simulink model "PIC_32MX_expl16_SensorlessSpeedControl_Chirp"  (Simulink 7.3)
settings: Solver=FixedStepDiscrete  StartTime=0.0  StopTime=10.0  FixedStep=.002  RelTol=1e-3
undefined symbols (not defined in the file or in its folder): bits, Buffer, characters, contain, Cosine, DiscIntNeverNeededParam, full, is, OC_HW, OCmax, PWM, Receive, Sine, sl_helperblocks, slDataTypeAndScale, Timer3, uint, When
libraries: dsPICdrivers x8, simulink x7

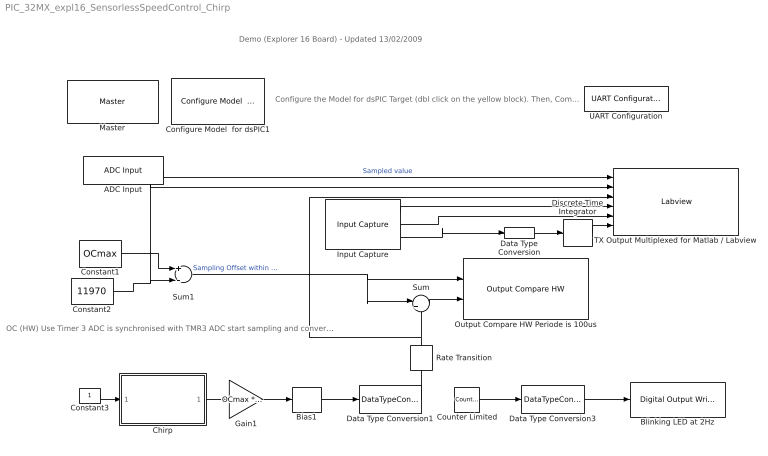
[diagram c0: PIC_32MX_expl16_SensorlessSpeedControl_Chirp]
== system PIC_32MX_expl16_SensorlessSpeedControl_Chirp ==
  note: Demo (Explorer 16 Board) - Updated 13/02/2009
  note: Configure the Model for dsPIC Target (dbl click on the yellow block). Then, Compile using the incremental build icon (second icon on right of the simulation mode (Normal))
  note: OC (HW) Use Timer 3 ADC is synchronised with TMR3 ADC start sampling and converting when TMR3 = OCmax (=PR3)
  ADC Input : dsPICdrivers/Peripheral I//O/ADC Input  Tag=dsPIC_ADC  Priority=5  ADC_TYPE=10 bits  ADC_MODE=Continuous sampling & get last channel value  NbrSampleStep=1  VoltRefpopup="AVdd  -  AVss"  OutFormatBitspopup=0000 00dd dddd dddd : Integer  InterruptPriority=6  ANCHANNELS=5  MaxName=ANmax = 1023  Rin=5e6  ADCS=29  SAMC=31  Temperature=25  DMAChannel=0  SampleTime=.002  Status="OK  |  Tsmp=4.844e-006 |  T/Channel=6.719e-006 |  Tall=6.719e-006"  SSRC=Timer3 (OC_HW PWM)
  Bias1 : Bias  Bias=floor(OCmax/2)
  Blinking LED at 2Hz : dsPICdrivers/Digital I//O/Digital Output Write  Tag=dsPIC_Digital_Output  Priority=5  PORT=A  Pin=[2]  Simultaneous=off  OrderingInOutPopup=None
  Chirp : Subsystem  mask{Fmax=15, Tend=60, Fs=500}
  Configure Model  for dsPIC1 : dsPICdrivers/Simulink Configuration/Configure Model  for dsPIC
  Constant1 : Constant  Value=OCmax  OutDataTypeMode=uint16  OutDataType=sfix(16)  OutScaling=2^0  OutDataTypeStr=uint16
  Constant2 : Constant  Value=11970  OutDataTypeMode=uint16  OutDataType=sfix(16)  OutScaling=2^0  OutDataTypeStr=uint16
  Constant3 : Constant  OutDataTypeMode=uint16  OutDataType=sfix(16)  OutScaling=2^0  OutDataTypeStr=uint16
  Counter Limited : simulink/Sources/Counter Limited  SystemSampleTime=-1  uplimit=1  tsamp=.25
  Data Type Conversion : DataTypeConversion  OutDataTypeMode=uint16  OutDataType=sfix(16)  OutScaling=2^0  OutDataTypeStr=uint16
  Data Type Conversion1 : DataTypeConversion  OutDataTypeMode=uint16  OutDataType=sfix(16)  OutScaling=2^0  OutDataTypeStr=uint16
  Data Type Conversion3 : DataTypeConversion  OutDataTypeMode=boolean  OutDataType=sfix(16)  OutScaling=2^0  OutDataTypeStr=boolean
  Discrete-Time Integrator : DiscreteIntegrator  gainval=500  SampleTime=-1  OutDataTypeMode=uint16  OutDataType=sfix(16)  OutScaling=2^0  OutDataTypeStr=uint16  ICPrevOutput=DiscIntNeverNeededParam  ICPrevScaledInput=DiscIntNeverNeededParam
  Gain1 : Gain  Gain=OCmax *.3  ParameterDataType=sfix(16)  ParameterScaling=2^0  OutDataTypeMode=int16  OutDataType=sfix(16)  OutScaling=2^0  OutDataTypeStr=int16
  Input Capture : dsPICdrivers/Peripheral I//O/Input Capture  Tag=dsPIC_PWM_IC  Priority=5  IntPriority=7  Channel=[1 ]  Channel_UP_Down_Periode=[3]  MaxChannel=[0.15]  SafeMarge=[10]  MaxName=' IC1max '  Precision=[15.917]  Timer=[2]  ChangeDetected=[1]  ChangeDetectedPortRef=3  SampleTime=-1  Status=OK
  Master : dsPICdrivers/Master  Tag=dsPIC_MASTER  Priority=1  TimeStepType=Timer1  picType=32MX460F512L  fcy=96000000  Quartz_33f=8e6  PLLActive_33f=on  fcyDesired_33f=96e6  tmr1="[8  23999  0]"  tmr1Info="Time Step : 0.002  ;   Error : 0%  PR1=23999"  tmr2345="[256    8    0    0]"  tmr2345cfg=[-1 -1 -1 -1]  IOautoConf=on  typePort="[ 0   0  10   0   0   0   0   0   0   0   0   0   0   0   0   0   0   0   0   0   0   8   0   0   0   0   0   0   0   0   0   0   0   0   0   0   0   0   0   0   0   0   0   0   0   0   0   0  24   0   0   0   0   0   0   0   6   0   0   0   0   0   0   0   0   0   0   0   0   0   0   0   0   0   0   0   0   0   0   0   0   0   0   0   4   5   0   0   0   0   0   0   0   0   0   0   0   0   0   0 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"  TRIS="[ 65531  65535  65535  65534  65535  65535  65535 ]"  ADPCFG=0  MasterBusyPort=None  MasterOverloadPort=None  FOSC=Quartz (XT - HS)  ClockSwitchMonitor=Both disabled  TempProtection_33f=TEMP_ON  FPBOR=<empty>  PWRT=disable  MCLR=<empty>  PowerSave=off  OverrideFcy=off  NewFcy=1e6  PR2345="[65535  11999  65535  65535]"
  Output Compare HW Periode is 100us : dsPICdrivers/Peripheral I//O/Output Compare HW  Tag=dsPIC_OC_HW_out  Priority=5  OC_Mode=PWM Time Set-Reset (glitch possible)  Timer=3  CHANNEL=[1 ]  Channel_UP_Down_Periode=[16]  PeriodeInput=off  MaxChannel=0.001  MaxName=' OCmax '  Precision=[13.5507]  Status=OK  SafeMarge=[0]  PortLetter=[68]  PortNumber=[0]  MaxValues=[11999]  NPORTS=2
  Rate Transition : RateTransition  Integrity=off
  Sum : Sum  Inputs=|++  OutDataType=sfix(16)  OutScaling=2^0
  Sum1 : Sum  Inputs=+-  OutDataType=sfix(16)  OutScaling=2^0
  TX Output Multiplexed for Matlab / Labview : dsPICdrivers/Serial PORT/TX Output Multiplexed for Matlab // Labview  Tag=dsPIC_TX_Multiplexed  Priority=5  UART=2  CleverSpreadingChk=on  CleverSpreading=1  CHANNEL=[0 1 2 3 4 5]  CHANNELBLOCKED=[]  CHANNELBLOCKED_BITEWISE=0  Status=OK
  UART Configuration : dsPICdrivers/Serial PORT/UART Configuration  Tag=dsPIC_config_UART  Priority=2  UART=2  proposed_BAUD=115200  ALT_TX_RX=on  InterruptTxWhen=When Transmit Buffer is empty  TXInterruptPri=1  TxBufferSize=32  TXEN=on  InterruptRxWhen=When Receive Buffer is full (contain 4 characters)  RXInterruptPri=2  RxBufferSize=32  BAUD=115200  UxBRG=51  Info="UxBRG = 51   ||  Real Baud : 115385   ||  % error : 0.16026  ||  max 23.0769 Bytes / Step"  RealBaud=0
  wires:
  Counter Limited/1 -> Data Type Conversion3/1
  ADC Input/1 -> TX Output Multiplexed for Matlab / Labview/1  "Sampled value"
  Sum/1 -> Output Compare HW Periode is 100us/2
  Sum1/1 -> Output Compare HW Periode is 100us/1, Sum/1  "Sampling Offset within PWM"
  Constant1/1 -> Sum1/1
  Data Type Conversion3/1 -> Blinking LED at 2Hz/1
  Rate Transition/1 -> Sum/2, TX Output Multiplexed for Matlab / Labview/3
  Input Capture/1 -> TX Output Multiplexed for Matlab / Labview/4
  Input Capture/2 -> TX Output Multiplexed for Matlab / Labview/5
  Input Capture/3 -> Data Type Conversion/1
  Discrete-Time Integrator/1 -> TX Output Multiplexed for Matlab / Labview/6
  Data Type Conversion/1 -> Discrete-Time Integrator/1
  Constant2/1 -> Sum1/2, TX Output Multiplexed for Matlab / Labview/2
  Data Type Conversion1/1 -> Rate Transition/1
  Constant3/1 -> Chirp/1(Enable =1 Stop = 0)
  Chirp/1(Chirp) -> Gain1/1
  Gain1/1 -> Bias1/1
  Bias1/1 -> Data Type Conversion1/1

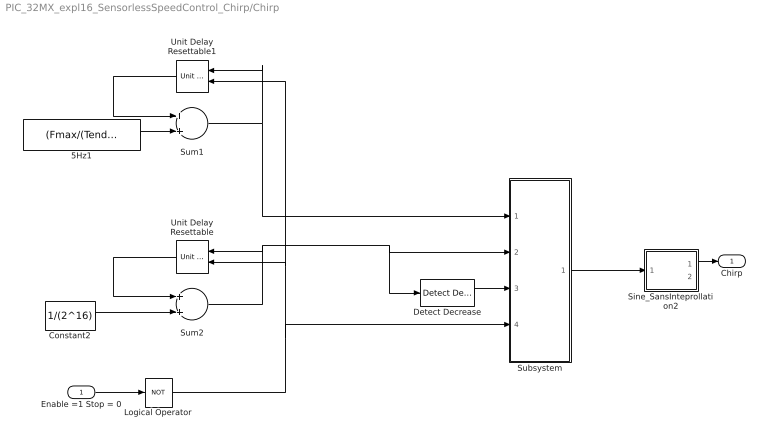
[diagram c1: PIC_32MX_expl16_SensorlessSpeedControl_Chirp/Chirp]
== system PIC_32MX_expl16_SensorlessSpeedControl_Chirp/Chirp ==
  Enable =1 Stop = 0 : Inport
  5Hz1 : Constant  Value=(Fmax/(Tend*2))/((1/2^16)*Fs)*(1/Fs)  OutDataTypeMode=Specify via dialog  OutDataType=fixdt(0,32,16)  ConRadixGroup=Best Precision: Vector-wise  OutDataTypeStr=fixdt(0,32,16)  SampleTime=1/Fs
  Constant2 : Constant  Value=1/(2^16)  OutDataType=sfix(16)  OutScaling=2^0  OutDataTypeStr=Inherit: Inherit via back propagation  SampleTime=1/Fs
  Detect Decrease : simulink/Logic and Bit Operations/Detect Decrease  SystemSampleTime=-1  vinit=0.0
  Logical Operator : Logic  Operator=NOT  AllPortsSameDT=off  OutDataTypeMode=boolean  OutDataTypeStr=boolean
  Sine_SansInteprollation2 : Subsystem  TreatAsAtomicUnit=on  mask(Sine and Cosine){Formula=sin(2*pi*u) and cos(2*pi*u), NumDataPoints=(2^13)+1, OutputWordLength=16}
      mask prompts: Formula "Output formula"; NumDataPoints "Number of data points for lookup table:"; OutputWordLength "Output word length:"
      mask help: Implement sine and cosine functions in fixed point using a lookup table approach that exploits quarter wave symmetry. The output fraction length equals the output word length minus 2. The most efficient implementation is obtained when the number of data points is (2^n)+1 where n is an integer.
      mask init:
      | if (~isnumeric(OutputWordLength)) || ( length(OutputWordLength) > 1 ) || ( OutputWordLength < 2 ) || ( floor(OutputWordLength) ~= OutputWordLength )
      |     error(DAStudio.message('Simulink:blocks:SineLookupWordLengthTooSmall'));
      | end
      | if (~isnumeric(NumDataPoints)) || ( length(NumDataPoints) > 1 ) || ( NumDataPoints < 2 ) || ( floor(NumDataPoints) ~= NumDataPoints )
      |     error(DAStudio.message('Simulink:blocks:SineLookupNumDataPtsTooSmall'));
      | end
      | if ( 2^(OutputWordLength-2) + 1 ) < NumDataPoints
      |     smallEnoughNumDataPoints = ( 2^(OutputWordLength-2) + 1 );
      |     bigEnoughOutputWordLength = ceil(log2(NumDataPoints-1))+2;
      |     error(DAStudio.message('Simulink:blocks:SineLookupEitherTooSmall',...
      |         NumDataPoints, ...
      |         smallEnoughNumDataPoints, ...
      |         OutputWordLength, ...
      |         bigEnoughOutputWordLength));
      | end
      | slsincos(Formula);
  Subsystem : Subsystem
  Sum1 : Sum  OutDataType=fixdt(0,16,16)  OutDataTypeStr=Inherit: Inherit via back propagation
  Sum2 : Sum  OutDataTypeMode=Specify via dialog  OutDataType=fixdt(0,16,16)  OutDataTypeStr=fixdt(0,16,16)
  Unit Delay Resettable : simulink/Additional Math & Discrete/Additional Discrete/Unit Delay Resettable  SystemSampleTime=-1  vinit=0.0  tsamp=-1
  Unit Delay Resettable1 : simulink/Additional Math & Discrete/Additional Discrete/Unit Delay Resettable  SystemSampleTime=-1  vinit=0.0  tsamp=-1
  Chirp : Outport
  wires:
  Sum2/1 -> Detect Decrease/1, Subsystem/2(Compteur), Unit Delay Resettable/1
  Unit Delay Resettable/1 -> Sum2/1
  Constant2/1 -> Sum2/2
  Subsystem/1(Out1) -> Sine_SansInteprollation2/1(u)
  Detect Decrease/1 -> Subsystem/3(Trig)
  Logical Operator/1 -> Subsystem/4(Reset), Unit Delay Resettable/2, Unit Delay Resettable1/2
  Sum1/1 -> Unit Delay Resettable1/1, Subsystem/1(Frequence)
  Unit Delay Resettable1/1 -> Sum1/1
  5Hz1/1 -> Sum1/2
  Sine_SansInteprollation2/1(sin(2*pi*u)) -> Chirp/1
  Enable =1 Stop = 0/1 -> Logical Operator/1

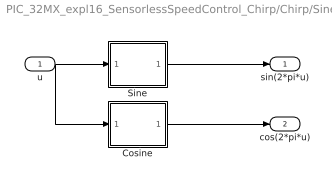
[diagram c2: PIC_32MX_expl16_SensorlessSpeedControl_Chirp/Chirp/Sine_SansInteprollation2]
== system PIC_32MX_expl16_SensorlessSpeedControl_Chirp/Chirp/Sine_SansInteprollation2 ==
  u : Inport  OutDataType=sfix(16)  OutScaling=2^0
  Cosine : Subsystem  AncestorBlock=sl_helperblocks/Cosine  mask(Cosine){NumDataPoints=NumDataPoints, OutputWordLength=OutputWordLength}
      mask prompts: NumDataPoints "Number of data points for lookup table:"; OutputWordLength "Output word length:"
      mask help: Implement a Cosine function in Fixed-Point using a lookup table approach that exploits quarter wave symmetry. The output fraction length equals output word length minus 2. The most efficient implementation is obtained when the number of data points is a power of 2 plus 1. For example, (2^5)+1.
      mask init:
      | XData = linspace(0,0.25,NumDataPoints);
      | %
      | % using sin for the data is not a mistake.
      | % parameter pooling will cause the data for similar sines and cosines to
      | % be shared.  This can save significant amounts of ROM.
      | %
      | YData = sin(2*pi*XData);
      | OutputFracLength = OutputWordLength-2;
  Sine : Subsystem  AncestorBlock=sl_helperblocks/Sine  mask(Sine){NumDataPoints=NumDataPoints, OutputWordLength=OutputWordLength}
      mask prompts: NumDataPoints "Number of data points for lookup table:"; OutputWordLength "Output word length:"
      mask help: Implement a Sine function in Fixed-Point using a lookup table approach that exploits quarter wave symmetry. The output fraction length equals output word length minus 2. The most efficient implementation is obtained when the number of data points is a power of 2 plus 1. For example, (2^5)+1.
      mask init:
      | XData = linspace(0,0.25,NumDataPoints);
      | YData = sin(2*pi*XData);
      | OutputFracLength = OutputWordLength-2;
  sin(2*pi*u) : Outport  OutDataType=sfix(16)  OutScaling=2^0
  cos(2*pi*u) : Outport  Port=2
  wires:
  u/1 -> Sine/1(In1), Cosine/1(In1)
  Sine/1(y) -> sin(2*pi*u)/1
  Cosine/1(y) -> cos(2*pi*u)/1

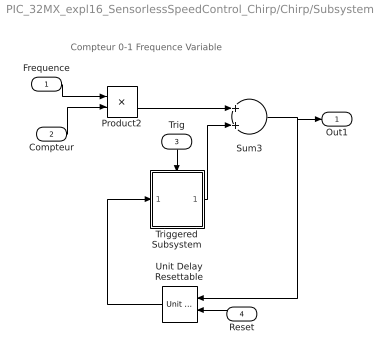
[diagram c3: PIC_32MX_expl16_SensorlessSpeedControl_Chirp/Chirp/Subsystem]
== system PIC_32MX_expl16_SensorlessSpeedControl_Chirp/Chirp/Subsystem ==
  note: Compteur 0-1 Frequence Variable
  Frequence : Inport
  Compteur : Inport  Port=2
  Trig : Inport  Port=3
  Reset : Inport  Port=4
  Product2 : Product  OutDataTypeMode=Specify via dialog  OutDataType=fixdt(0,16,16)  OutDataTypeStr=fixdt(0,16,16)
  Sum3 : Sum  OutDataTypeMode=Specify via dialog  OutDataType=fixdt(0,16,16)  OutDataTypeStr=fixdt(0,16,16)
  Triggered Subsystem : Subsystem  TreatAsAtomicUnit=on
  Unit Delay Resettable : simulink/Additional Math & Discrete/Additional Discrete/Unit Delay Resettable  SystemSampleTime=-1  vinit=0.0  tsamp=-1
  Out1 : Outport
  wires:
  Product2/1 -> Sum3/1
  Triggered Subsystem/1(Out1) -> Sum3/2
  Unit Delay Resettable/1 -> Triggered Subsystem/1(In1)
  Sum3/1 -> Out1/1, Unit Delay Resettable/1
  Compteur/1 -> Product2/2
  Frequence/1 -> Product2/1
  Trig/1 -> Triggered Subsystem/Trigger
  Reset/1 -> Unit Delay Resettable/2

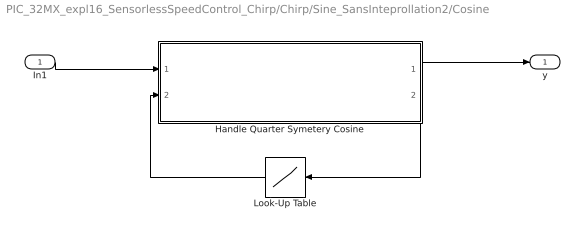
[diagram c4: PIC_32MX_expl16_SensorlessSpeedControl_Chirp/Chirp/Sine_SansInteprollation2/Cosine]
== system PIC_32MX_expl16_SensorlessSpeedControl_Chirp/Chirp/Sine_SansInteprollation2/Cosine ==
  In1 : Inport  OutDataType=sfix(16)  OutScaling=2^0
  Handle Quarter Symetery Cosine : Subsystem
  Look-Up Table : Lookup  InputValues=XData  Table=YData  LookUpMeth=Use Input Nearest  OutDataTypeMode=Specify via dialog  OutDataType=slDataTypeAndScale(('sfix(OutputWordLength)'),('2^-OutputFracLength'))  OutDataTypeStr=slDataTypeAndScale(('sfix(OutputWordLength)'),('2^-OutputFracLength'))
  y : Outport  OutDataType=sfix(16)  OutScaling=2^0
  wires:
  Handle Quarter Symetery Cosine/2(Input To Lookup Table) -> Look-Up Table/1
  Look-Up Table/1 -> Handle Quarter Symetery Cosine/2(Output From Lookup Table)
  In1/1 -> Handle Quarter Symetery Cosine/1(Raw Angle)
  Handle Quarter Symetery Cosine/1(Cosine) -> y/1

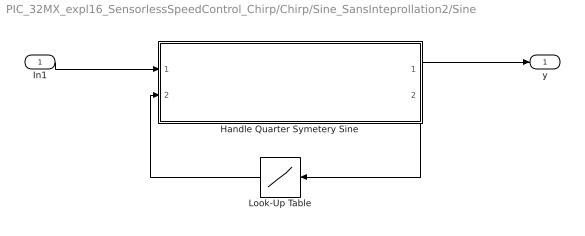
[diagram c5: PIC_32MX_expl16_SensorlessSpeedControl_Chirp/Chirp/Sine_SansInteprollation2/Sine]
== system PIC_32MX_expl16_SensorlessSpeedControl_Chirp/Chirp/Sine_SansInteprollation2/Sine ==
  In1 : Inport  OutDataType=sfix(16)  OutScaling=2^0
  Handle Quarter Symetery Sine : Subsystem
  Look-Up Table : Lookup  InputValues=XData  Table=YData  LookUpMeth=Use Input Nearest  OutDataTypeMode=Specify via dialog  OutDataType=slDataTypeAndScale(('sfix(OutputWordLength)'),('2^-OutputFracLength'))  OutDataTypeStr=slDataTypeAndScale(('sfix(OutputWordLength)'),('2^-OutputFracLength'))
  y : Outport  OutDataType=sfix(16)  OutScaling=2^0
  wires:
  Handle Quarter Symetery Sine/1(Sine) -> y/1
  In1/1 -> Handle Quarter Symetery Sine/1(Raw Angle)
  Look-Up Table/1 -> Handle Quarter Symetery Sine/2(Output From Lookup Table)
  Handle Quarter Symetery Sine/2(Input To Lookup Table) -> Look-Up Table/1

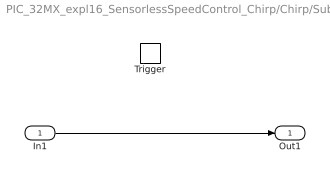
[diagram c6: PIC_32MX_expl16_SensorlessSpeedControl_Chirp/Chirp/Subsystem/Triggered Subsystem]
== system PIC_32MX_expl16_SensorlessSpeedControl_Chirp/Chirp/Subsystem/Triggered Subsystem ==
  In1 : Inport  OutDataType=sfix(16)  OutScaling=2^0
  Trigger : TriggerPort
  Out1 : Outport  OutDataType=sfix(16)  OutScaling=2^0
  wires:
  In1/1 -> Out1/1

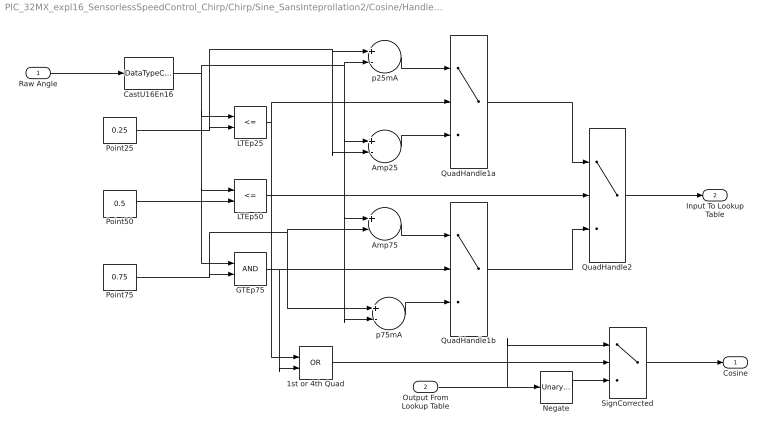
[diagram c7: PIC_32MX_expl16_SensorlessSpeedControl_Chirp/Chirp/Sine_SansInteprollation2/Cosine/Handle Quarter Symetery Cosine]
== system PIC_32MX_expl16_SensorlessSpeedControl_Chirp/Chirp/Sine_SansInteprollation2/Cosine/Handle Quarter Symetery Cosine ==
  Raw Angle : Inport  OutDataType=sfix(16)  OutScaling=2^0
  Output From Lookup Table : Inport  Port=2  OutDataType=sfix(16)  OutScaling=2^0
  1st or 4th Quad : Logic  Operator=OR  AllPortsSameDT=off  OutDataTypeMode=Specify via dialog  OutDataTypeStr=uint(8)
  Amp25 : Sum  Inputs=+-  OutDataType=uint(8)  OutScaling=1
  Amp75 : Sum  Inputs=+-  OutDataType=uint(8)  OutScaling=1
  CastU16En16 : DataTypeConversion  OutDataTypeMode=Specify via dialog  OutDataType=slDataTypeAndScale(('ufix(OutputWordLength)'),('2^-OutputWordLength'))  OutDataTypeStr=slDataTypeAndScale(('ufix(OutputWordLength)'),('2^-OutputWordLength'))
  GTEp75 : RelationalOperator  LogicOutDataTypeMode=Specify via dialog  OutDataTypeStr=uint(8)  ZeroCross=off
  LTEp25 : RelationalOperator  Operator=<=  LogicOutDataTypeMode=Specify via dialog  OutDataTypeStr=uint(8)  ZeroCross=off
  LTEp50 : RelationalOperator  Operator=<=  LogicOutDataTypeMode=Specify via dialog  OutDataTypeStr=uint(8)  ZeroCross=off
  Negate : simulink/Math Operations/Unary Minus  DoSatur=off
  Point25 : Constant  Value=0.25  OutDataTypeMode=Specify via dialog  OutDataType=slDataTypeAndScale(('ufix(OutputWordLength)'),('2^-OutputWordLength'))  ConRadixGroup=Best Precision: Vector-wise  OutDataTypeStr=slDataTypeAndScale(('ufix(OutputWordLength)'),('2^-OutputWordLength'))
  Point50 : Constant  Value=0.5  OutDataTypeMode=Specify via dialog  OutDataType=slDataTypeAndScale(('ufix(OutputWordLength) '),('2^-OutputWordLength'))  ConRadixGroup=Best Precision: Vector-wise  OutDataTypeStr=slDataTypeAndScale(('ufix(OutputWordLength) '),('2^-OutputWordLength'))
  Point75 : Constant  Value=0.75  OutDataTypeMode=Specify via dialog  OutDataType=slDataTypeAndScale(('ufix(OutputWordLength) '),('2^-OutputWordLength'))  ConRadixGroup=Best Precision: Vector-wise  OutDataTypeStr=slDataTypeAndScale(('ufix(OutputWordLength) '),('2^-OutputWordLength'))
  QuadHandle1a : Switch  Criteria=u2 ~= 0  ZeroCross=off
  QuadHandle1b : Switch  Criteria=u2 ~= 0  ZeroCross=off
  QuadHandle2 : Switch  Criteria=u2 ~= 0  ZeroCross=off
  SignCorrected : Switch  Threshold=1  ZeroCross=off
  p25mA : Sum  Inputs=+-  OutDataType=uint(8)  OutScaling=1
  p75mA : Sum  Inputs=+-  OutDataType=uint(8)  OutScaling=1
  Cosine : Outport  OutDataType=sfix(16)  OutScaling=2^0
  Input To Lookup Table : Outport  Port=2  OutDataType=sfix(16)  OutScaling=2^0
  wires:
  1st or 4th Quad/1 -> SignCorrected/2
  QuadHandle2/1 -> Input To Lookup Table/1
  QuadHandle1b/1 -> QuadHandle2/3
  QuadHandle1a/1 -> QuadHandle2/1
  GTEp75/1 -> 1st or 4th Quad/2, QuadHandle1b/2
  p75mA/1 -> QuadHandle1b/3
  Amp75/1 -> QuadHandle1b/1
  LTEp25/1 -> 1st or 4th Quad/1, QuadHandle1a/2
  LTEp50/1 -> QuadHandle2/2
  Amp25/1 -> QuadHandle1a/3
  Point50/1 -> LTEp50/2
  p25mA/1 -> QuadHandle1a/1
  Point75/1 -> p75mA/1, Amp75/2, GTEp75/2
  CastU16En16/1 -> p75mA/2, Amp75/1, Amp25/1, p25mA/2, GTEp75/1, LTEp50/1, LTEp25/1
  Negate/1 -> SignCorrected/3
  SignCorrected/1 -> Cosine/1
  Output From Lookup Table/1 -> SignCorrected/1, Negate/1
  Point25/1 -> Amp25/2, p25mA/1, LTEp25/2
  Raw Angle/1 -> CastU16En16/1

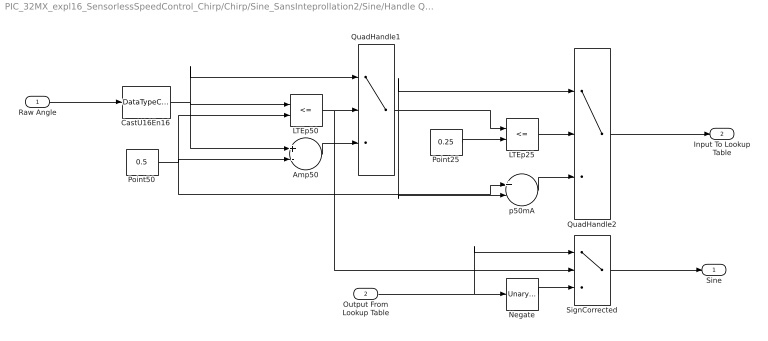
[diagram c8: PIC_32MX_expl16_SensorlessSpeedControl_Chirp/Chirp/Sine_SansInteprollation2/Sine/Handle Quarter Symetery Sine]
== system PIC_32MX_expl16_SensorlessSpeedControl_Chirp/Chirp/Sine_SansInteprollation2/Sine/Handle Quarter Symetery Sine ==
  Raw Angle : Inport  OutDataType=sfix(16)  OutScaling=2^0
  Output From Lookup Table : Inport  Port=2  OutDataType=sfix(16)  OutScaling=2^0
  Amp50 : Sum  Inputs=+-  OutDataType=uint(8)  OutScaling=1
  CastU16En16 : DataTypeConversion  OutDataTypeMode=Specify via dialog  OutDataType=slDataTypeAndScale(('ufix(OutputWordLength)'),('2^-OutputWordLength'))  OutDataTypeStr=slDataTypeAndScale(('ufix(OutputWordLength)'),('2^-OutputWordLength'))
  LTEp25 : RelationalOperator  Operator=<=  LogicOutDataTypeMode=Specify via dialog  OutDataTypeStr=uint(8)  ZeroCross=off
  LTEp50 : RelationalOperator  Operator=<=  LogicOutDataTypeMode=Specify via dialog  OutDataTypeStr=uint(8)  ZeroCross=off
  Negate : simulink/Math Operations/Unary Minus  DoSatur=off
  Point25 : Constant  Value=0.25  OutDataTypeMode=Specify via dialog  OutDataType=slDataTypeAndScale(('ufix(OutputWordLength)'),('2^-OutputWordLength'))  ConRadixGroup=Best Precision: Vector-wise  OutDataTypeStr=slDataTypeAndScale(('ufix(OutputWordLength)'),('2^-OutputWordLength'))
  Point50 : Constant  Value=0.5  OutDataTypeMode=Specify via dialog  OutDataType=slDataTypeAndScale(('ufix(OutputWordLength) '),('2^-OutputWordLength'))  ConRadixGroup=Best Precision: Vector-wise  OutDataTypeStr=slDataTypeAndScale(('ufix(OutputWordLength) '),('2^-OutputWordLength'))
  QuadHandle1 : Switch  Criteria=u2 ~= 0  ZeroCross=off
  QuadHandle2 : Switch  Criteria=u2 ~= 0  ZeroCross=off
  SignCorrected : Switch  Threshold=1  ZeroCross=off
  p50mA : Sum  Inputs=+-  OutDataType=uint(8)  OutScaling=1
  Sine : Outport  OutDataType=sfix(16)  OutScaling=2^0
  Input To Lookup Table : Outport  Port=2  OutDataType=sfix(16)  OutScaling=2^0
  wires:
  Raw Angle/1 -> CastU16En16/1
  LTEp50/1 -> QuadHandle1/2, SignCorrected/2
  QuadHandle1/1 -> LTEp25/1, QuadHandle2/1, p50mA/2
  Point25/1 -> LTEp25/2
  LTEp25/1 -> QuadHandle2/2
  QuadHandle2/1 -> Input To Lookup Table/1
  CastU16En16/1 -> LTEp50/1, QuadHandle1/1, Amp50/1
  Output From Lookup Table/1 -> Negate/1, SignCorrected/1
  SignCorrected/1 -> Sine/1
  Amp50/1 -> QuadHandle1/3
  Negate/1 -> SignCorrected/3
  p50mA/1 -> QuadHandle2/3
  Point50/1 -> LTEp50/2, Amp50/2, p50mA/1
